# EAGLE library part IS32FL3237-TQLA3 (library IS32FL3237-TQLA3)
LED Lighting Drivers 36-Channel LED Driver, eTQFP-48 (9.0mm x 9.0mm) Source: Datasheet
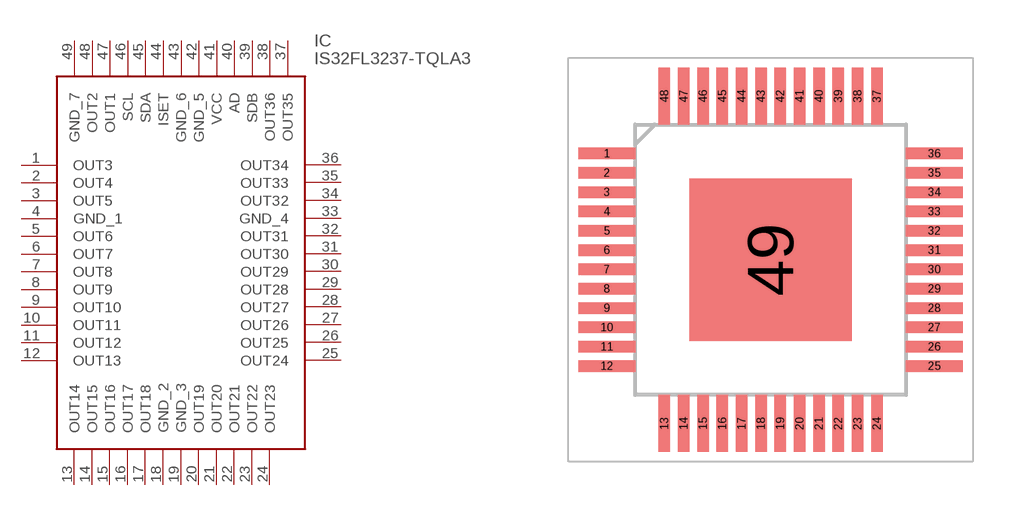
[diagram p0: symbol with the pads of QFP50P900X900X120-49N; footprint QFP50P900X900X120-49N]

Designator prefix IC

## IS32FL3237-TQLA3 (Description: LED Lighting Drivers 36-Channel LED Driver, eTQFP-48 (9.0mm x 9.0mm); Height: 1.2mm; Manufacturer_Name: Lumissil; Manufacturer_Part_Number: IS32FL3237-TQLA3)  [QFP50P900X900X120-49N]
1  OUT3
2  OUT4
3  OUT5
4  GND_1
5  OUT6
6  OUT7
7  OUT8
8  OUT9
9  OUT10
10  OUT11
11  OUT12
12  OUT13
13  OUT14
14  OUT15
15  OUT16
16  OUT17
17  OUT18
18  GND_2
19  GND_3
20  OUT19
21  OUT20
22  OUT21
23  OUT22
24  OUT23
25  OUT24
26  OUT25
27  OUT26
28  OUT27
29  OUT28
30  OUT29
31  OUT30
32  OUT31
33  GND_4
34  OUT32
35  OUT33
36  OUT34
37  OUT35
38  OUT36
39  SDB
40  AD
41  VCC
42  GND_5
43  GND_6
44  ISET
45  SDA
46  SCL
47  OUT1
48  OUT2
49  GND_7

## Footprint QFP50P900X900X120-49N (pad centres in mm)
eTQFP-48
smd 1.475 x 0.3: 1 -4.238,2.75; 2 -4.238,2.25; 3 -4.238,1.75; 4 -4.238,1.25; 5 -4.238,0.75; 6 -4.238,0.25; 7 -4.238,-0.25; 8 -4.238,-0.75; 9 -4.238,-1.25; 10 -4.238,-1.75; 11 -4.238,-2.25; 12 -4.238,-2.75; 25 4.238,-2.75; 26 4.238,-2.25; 27 4.238,-1.75; 28 4.238,-1.25; 29 4.238,-0.75; 30 4.238,-0.25; 31 4.238,0.25; 32 4.238,0.75; 33 4.238,1.25; 34 4.238,1.75; 35 4.238,2.25; 36 4.238,2.75
smd 0.3 x 1.475: 13 -2.75,-4.238; 14 -2.25,-4.238; 15 -1.75,-4.238; 16 -1.25,-4.238; 17 -0.75,-4.238; 18 -0.25,-4.238; 19 0.25,-4.238; 20 0.75,-4.238; 21 1.25,-4.238; 22 1.75,-4.238; 23 2.25,-4.238; 24 2.75,-4.238; 37 2.75,4.238; 38 2.25,4.238; 39 1.75,4.238; 40 1.25,4.238; 41 0.75,4.238; 42 0.25,4.238; 43 -0.25,4.238; 44 -0.75,4.238; 45 -1.25,4.238; 46 -1.75,4.238; 47 -2.25,4.238; 48 -2.75,4.238
smd 4.21 x 4.21: 49 0,0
